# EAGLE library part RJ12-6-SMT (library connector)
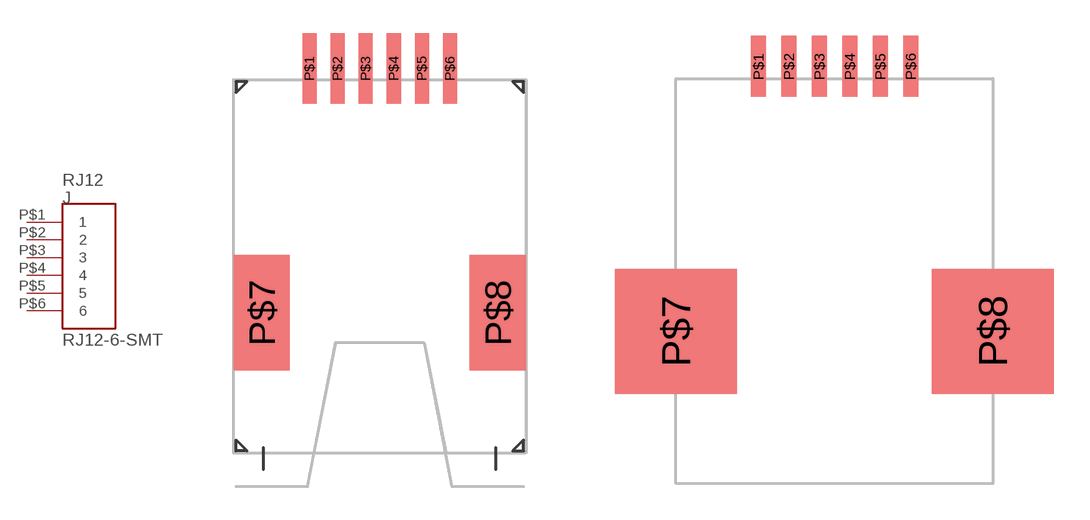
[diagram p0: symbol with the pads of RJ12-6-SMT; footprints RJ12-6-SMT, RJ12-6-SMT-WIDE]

Designator prefix J

## RJ12-6-SMT  [RJ12-6-SMT]
P$1  1
P$2  2
P$3  3
P$4  4
P$5  5
P$6  6

## RJ12-6-SMTWIDE  [RJ12-6-SMT-WIDE]
Pads as for RJ12-6-SMT

## RJ12-6-SMTTOP  [RJ12-6-SMT-TOPENTRY]
Pads as for RJ12-6-SMT

## RJ12-6-SMTNOSILK  [RJ12-6-SMT-NOSILK]
Pads as for RJ12-6-SMT

## Footprint RJ12-6-SMT (pad centres in mm)
smd 0.635 x 3.175: P$1 -3.175,17.399; P$2 -1.905,17.399; P$3 -0.635,17.399; P$4 0.635,17.399; P$5 1.905,17.399; P$6 3.175,17.399
smd 2.54 x 5.207: P$7 -5.334,6.35; P$8 5.334,6.35

## Footprint RJ12-6-SMT-WIDE (pad centres in mm)
smd 0.635 x 2.54: P$1 -3.175,17.399; P$2 -1.905,17.399; P$3 -0.635,17.399; P$4 0.635,17.399; P$5 1.905,17.399; P$6 3.175,17.399
smd 5.08 x 5.207: P$7 -6.604,6.35; P$8 6.604,6.35

## Footprint RJ12-6-SMT-TOPENTRY (pad centres in mm)
smd 0.76 x 5: P$1 -3.175,15.3; P$2 -1.905,15.3; P$3 -0.635,15.3; P$4 0.635,15.3; P$5 1.905,15.3; P$6 3.175,15.3
smd 8.8 x 4.5: P$7 0,-0.25

## Footprint RJ12-6-SMT-NOSILK (pad centres in mm)
smd 0.635 x 2.54: P$1 -3.175,17.399; P$2 -1.905,17.399; P$3 -0.635,17.399; P$4 0.635,17.399; P$5 1.905,17.399; P$6 3.175,17.399
smd 2.54 x 5.207: P$7 -5.334,6.35; P$8 5.334,6.35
